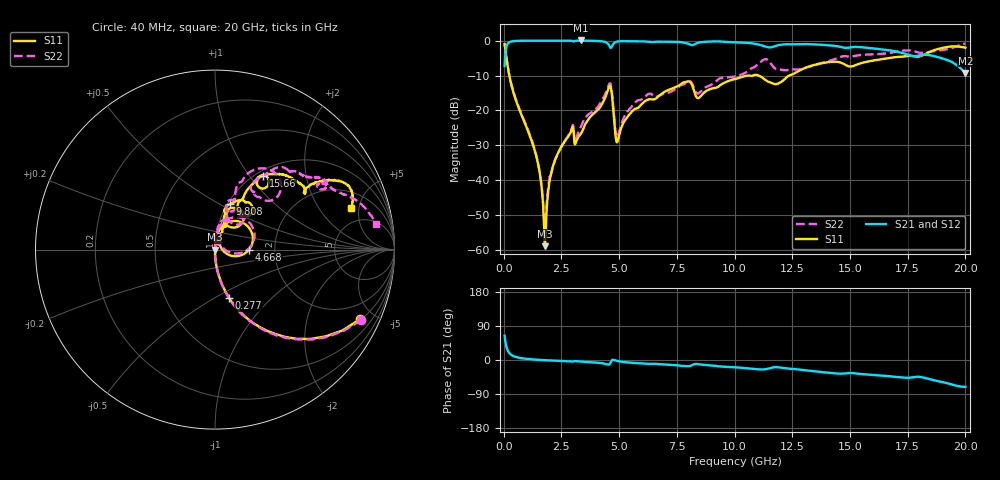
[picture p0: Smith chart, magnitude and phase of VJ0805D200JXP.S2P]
! VJ0805D200JXP
! DATE 10/29/2021  10:29
! CAPACITORS MOUNTED IN SERIES ON 25 MIL THICK MICROSTRIP SUBSTRATE
# GHz  S  MA  R  50.00
!  FREQ  S11M  S11A  S21M  S21A  S12M  S12A  S22M  S22A
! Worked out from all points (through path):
!   1601 points, 40 MHz to 20 GHz, reference 50 ohm
!   highest |S21| = 0.06 dB at 3.358 GHz (marker M1); lowest = -9.3 dB at 20 GHz (marker M2)
!   group delay of S21, straight-line fit = 9.03 ps
!   lowest |S11| = -59.0 dB at 1.786 GHz (marker M3), VSWR 1.00, Z = 50.1 - j0.0255 ohm
!   |S11| at or under -10 dB: 243 MHz to 10.62 GHz (10.37 GHz wide, 191 % of centre); 10.62 GHz to 10.8 GHz (177.5 MHz wide, 1.66 % of centre); 11.04 GHz to 12.36 GHz (1.313 GHz wide, 11.2 % of centre)
!   |S22| runs from -54.3 to -0.8 dB; largest |S21 - S12| = 0.0044
!   S11 on the Smith chart (normalised r, x): 40 MHz: 1.06, -4.11; 277 MHz: 1.00, -0.58; 4.668 GHz: 1.47, -0.00; 9.808 GHz: 1.03, +0.57; 15.66 GHz: 1.08, +1.17; 20 GHz: 3.27, +4.09
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0.04  0.8943 -25.8  0.4351 64.1  0.434 63.9  0.9036 -25.9
0.277025  0.2795 -73.8  0.9599 16.2  0.9592 16.2  0.2828 -73.9
1.41225  0.02186 -89.6  0.9994 0.9  0.9985 0.9  0.02265 -85.5
1.7865  0.001128 -13.0  0.9992 -0.5  0.9981 -0.5  0.001919 6.3
2.036  0.01184 90.7  0.9986 -1.3  0.9977 -1.3  0.01148 74.4
2.273025  0.02137 89.4  0.9991 -1.9  0.9979 -1.9  0.02105 81.6
2.921725  0.05 79.8  0.996 -3.8  0.9953 -3.9  0.0524 85.1
3.35835  0.04697 90.0  1.007 -4.3  1.005 -4.4  0.0595 96.4
3.370825  0.04783 91.0  1.006 -4.4  1.005 -4.5  0.0608 96.7
4.668225  0.1894 -0.0  0.8043 -2.2  0.8034 -2.3  0.2052 6.6
4.9302  0.03575 35.9  0.9727 -2.7  0.9721 -2.7  0.04123 43.7
5.716125  0.106 67.4  0.9807 -8.0  0.9799 -8.1  0.1317 82.1
6.70165  0.1588 71.8  0.9679 -10.6  0.9675 -10.6  0.1602 70.9
7.9741  0.2604 60.2  0.9072 -16.3  0.9062 -16.3  0.2589 60.2
8.44815  0.1505 63.8  0.941 -11.0  0.9392 -11.0  0.1762 61.1
9.807925  0.2688 71.6  0.9538 -18.6  0.9527 -18.6  0.3007 68.7
10.02  0.2806 68.6  0.947 -19.2  0.9459 -19.3  0.3065 69.0
11.49205  0.2555 46.1  0.8012 -22.3  0.7995 -22.4  0.5117 43.8
13.35083  0.4387 59.5  0.8879 -29.0  0.8866 -29.0  0.4351 60.2
15.6587  0.4918 56.8  0.7955 -38.0  0.7955 -38.0  0.6305 43.0
16.68165  0.5631 48.1  0.7284 -42.7  0.7283 -42.7  0.6626 37.4
20  0.7913 17.2  0.343 -70.9  0.3422 -71.2  0.9079 9.0
